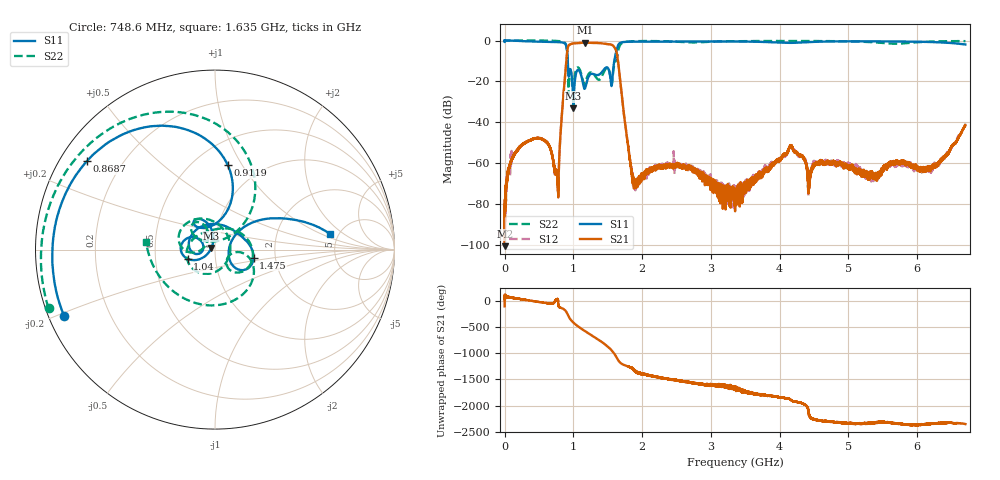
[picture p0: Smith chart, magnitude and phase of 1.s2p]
!Keysight Technologies,N5232A,MY52221221,A.10.65.11
!Date: Wednesday, December 06, 2023 14:48:53
!Correction: S11(Full 2 Port(1,4))
!S41(Full 2 Port(1,4))
!S14(Full 2 Port(1,4))
!S44(Full 2 Port(1,4))
!S2P File: Measurements: S11, S41, S14, S44:
# Hz S  RI  R 50
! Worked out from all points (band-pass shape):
!   16001 points, 300 kHz to 6.7 GHz, reference 50 ohm
!   highest |S21| = -1.00 dB at 1.168 GHz (marker M1); lowest = -100.7 dB at 3.65 MHz (marker M2)
!   |S21| within 3 dB of the highest: 916.5 MHz to 1.61 GHz (693.9 MHz wide, 54.9 % of centre)
!   lowest |S11| = -33.2 dB at 1.001 GHz (marker M3), VSWR 1.04, Z = 48 + j0.833 ohm
!   |S11| at or under -10 dB: 918.6 MHz to 1.595 GHz (676 MHz wide, 53.8 % of centre)
!   |S22| runs from -26.7 to 0.0 dB; largest |S21 - S12| = 0.0081
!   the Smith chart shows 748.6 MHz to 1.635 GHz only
!   S11 on the Smith chart (normalised r, x): 748.6 MHz: 0.04, -0.21; 868.7 MHz: 0.08, +0.31; 911.9 MHz: 0.71, +0.87; 1.04 GHz: 0.73, -0.08; 1.475 GHz: 1.54, -0.14; 1.635 GHz: 4.23, +1.28
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300000  1.003 -0.00232  -2e-05 -0.00012  -2.89e-05 -5.49e-05  1.002 -0.0017
3649850  1.001 -0.0126  8.73e-06 2.97e-06  6.3e-05 1.44e-05  0.9995 -0.0122
3.52453e8  0.3265 -0.8977  0.00337 0.000844  0.00344 0.000869  0.3628 -0.9343
7.485727e8  -0.8401 -0.3718  0.000549 0.0003  0.000562 0.000197  -0.927 -0.3277
8.687486e8  -0.7133 0.4934  -0.0802 -0.0257  -0.08 -0.0248  -0.6423 0.6356
9.118779e8  0.0705 0.4713  -0.2625 0.4913  -0.2621 0.4923  0.2196 0.4025
1.000649e9  -0.0201 0.00867  0.5389 -0.6628  0.5386 -0.6626  -0.0629 0.0102
1.040428e9  -0.1524 -0.0513  -0.0945 -0.8516  -0.0984 -0.8521  -0.1949 0.0275
1.117056e9  -0.1143 0.0682  -0.8636 -0.1658  -0.8654 -0.1659  0.00925 0.1476
1.167723e9  -0.0663 0.00107  -0.7437 0.4902  -0.741 0.4866  0.0763 -0.0431
1.338565e9  0.0127 0.1417  0.8682 0.0756  0.8712 0.0766  -0.0847 0.085
1.474653e9  0.2146 -0.0445  -0.4518 -0.6926  -0.4504 -0.6897  0.2074 0.00456
1.571798e9  0.1174 0.0861  -0.2958 0.7028  -0.2974 0.7022  0.1327 -0.0138
1.635446e9  0.639 0.0882  0.433 -0.1086  0.439 -0.1123  -0.3842 0.0426
1.721704e9  0.6135 -0.6789  -0.0168 -0.0173  -0.0165 -0.017  0.8851 -0.0703
1.88166e9  0.0255 -0.9381  -9.46e-05 0.000291  -0.000184 0.000279  0.3411 -0.8985
2.233812e9  -0.5749 -0.7439  0.000733 -0.000204  0.000844 -0.000152  -0.4863 -0.8339
3.35015e9  -0.948 -0.00946  -0.000111 9.16e-05  -0.000223 8.05e-05  -0.9632 -0.0523
4.159139e9  -0.8308 0.2803  0.000169 -0.00267  5.6e-06 -0.00251  -0.8936 0.3849
4.466906e9  -0.8449 0.3693  6.9e-05 -0.000738  0.00019 -0.000738  -0.8241 0.5141
5.583662e9  -0.4597 0.8313  -0.000989 -0.000231  -0.000842 -0.000121  -0.4281 0.7317
6.7e9  0.7719 0.2079  -0.00818 0.002  -0.00876 0.00155  -0.1224 0.9579
